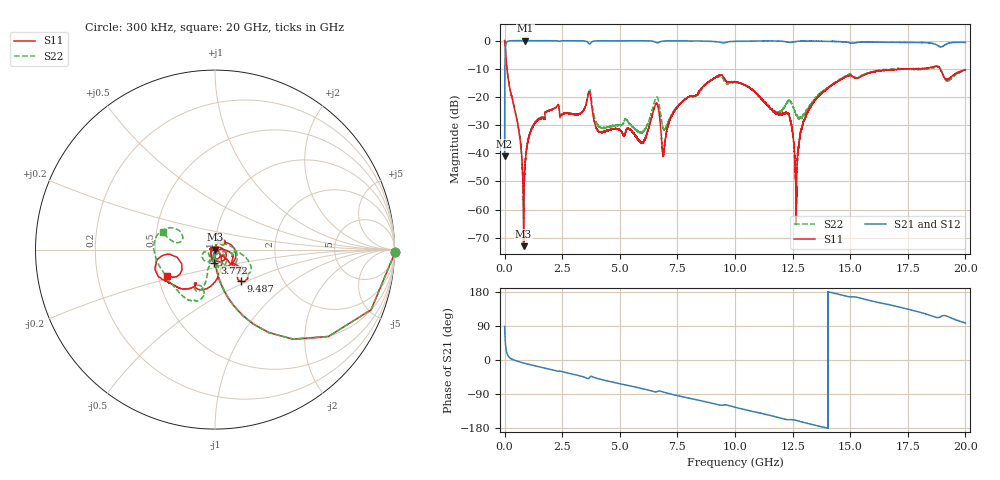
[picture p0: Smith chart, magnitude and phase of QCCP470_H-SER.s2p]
!{QCCP470}
!Johanson Technology Inc.
!www.johansontechnology.com
!Test Board Conditions:
!Substrate Type  RO4350B
!Substrate Thickness  20 mil
!Substrate Dk  3.66
!TL Type: GCPW
!TL Trace Width  36 mil
!TL Gap  12 mil
!Electrode orientation  Horizontal
!DUT TOPOLOGY	SERIES
!Mounting Pad LxW  26x36 mil
# MHz S  dB  R 50
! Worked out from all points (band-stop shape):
!   20001 points, 300 kHz to 20 GHz, reference 50 ohm
!   highest |S21| = -0.01 dB at 893.3 MHz (marker M1); lowest = -41.2 dB at 300 kHz (marker M2)
!   |S21| within 3 dB of the highest: 34.82 MHz to end of sweep
!   lowest |S11| = -73.0 dB at 824.3 MHz (marker M3), VSWR 1.00, Z = 50 - j0.0189 ohm
!   |S11| at or under -10 dB: 102.6 MHz to 17.5 GHz (17.4 GHz wide, 198 % of centre); 17.50459 GHz to 17.57685 GHz (72.26 MHz wide, 0.412 % of centre); 18.9 GHz to end of sweep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
!   |S22| runs from -63.2 to 0.0 dB; largest |S21 - S12| = 0.018
!   S11 on the Smith chart (normalised r, x): 300 kHz: open; 3.772 GHz: 0.98, -0.15; 9.487 GHz: 1.25, -0.46; 20 GHz: 0.56, -0.18
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0.3  0.03 -0.9  -41.16 88.7  -41.16 89.0  0.04 -0.8
122.298  -11.44 -75.5  -0.35 14.3  -0.34 14.2  -11.42 -75.4
824.288  -73.00 -57.6  -0.01 -8.0  -0.01 -8.1  -59.58 -24.5
893.287  -43.59 78.8  -0.01 -9.1  -0.01 -9.2  -43.61 68.2
1045.284  -34.49 78.7  -0.02 -11.4  -0.02 -11.5  -34.46 74.3
1384.279  -28.66 72.6  -0.03 -16.3  -0.03 -16.3  -28.46 71.2
3334.25  -25.71 46.7  -0.10 -43.0  -0.09 -43.0  -25.60 37.3
3772.243  -22.57 -93.2  -0.56 -43.1  -0.56 -43.1  -21.11 -86.2
4148.238  -32.44 -166.7  -0.09 -50.8  -0.08 -50.7  -30.81 -102.3
5939.211  -36.26 96.3  -0.07 -75.0  -0.06 -75.0  -32.82 -70.8
6667.2  -23.79 -81.5  -0.73 -82.3  -0.73 -82.2  -20.95 -81.9
6906.196  -40.04 -29.3  -0.16 -84.9  -0.17 -84.9  -31.51 -67.4
7514.187  -23.43 -5.4  -0.09 -94.1  -0.10 -94.1  -23.29 -9.7
9487.158  -12.81 -50.3  -0.87 -119.1  -0.86 -119.1  -13.59 -42.2
10000.15  -14.67 -39.0  -0.28 -124.8  -0.29 -124.7  -14.78 -33.8
11729.12  -25.22 -37.4  -0.13 -149.2  -0.14 -149.2  -25.35 -83.2
12289.12  -25.98 -91.7  -0.55 -157.5  -0.54 -157.3  -21.63 -129.6
12658.11  -62.78 32.2  -0.33 -159.4  -0.33 -159.5  -26.39 -167.3
12901.11  -31.09 -34.4  -0.20 -163.4  -0.18 -163.4  -27.58 -135.7
13334.1  -22.81 -60.2  -0.18 -170.0  -0.17 -170.0  -22.08 -113.3
16667.05  -10.51 -137.1  -0.61 146.2  -0.70 146.1  -10.21 -112.7
20000  -10.33 -150.9  -0.67 97.6  -0.75 97.5  -10.25 161.3
